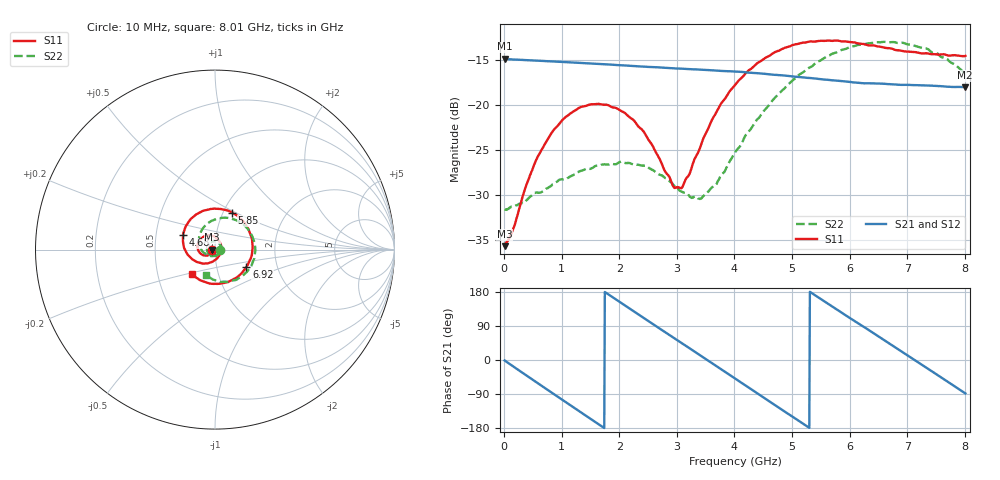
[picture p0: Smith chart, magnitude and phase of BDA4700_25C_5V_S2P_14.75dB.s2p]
!Agilent Technologies,E5071B,MY42404982,A.09.10
!Date: Mon Oct 20 13:33:35 2025
!Data & Calibration Information:
!Freq	S11:SOLT2(ON)	S21:SOLT2(ON)	S12:SOLT2(ON)	S22:SOLT2(ON)
# Hz S RI R 50
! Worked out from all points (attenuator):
!   801 points, 10 MHz to 8.01 GHz, reference 50 ohm
!   highest |S21| = -14.85 dB at 10 MHz (marker M1); lowest = -18.0 dB at 8 GHz (marker M2)
!   lowest |S11| = -35.7 dB at 10 MHz (marker M3), VSWR 1.03, Z = 48.4 - j0.117 ohm
!   |S11| at or under -10 dB: start of sweep to end of sweep
!   |S22| runs from -31.7 to -13.0 dB; largest |S21 - S12| = 0.0014
!   S11 on the Smith chart (normalised r, x): 10 MHz: 0.97, -0.00; 4.68 GHz: 0.69, +0.11; 5.85 GHz: 1.10, +0.48; 6.92 GHz: 1.39, -0.28; 8.01 GHz: 0.75, -0.21
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1e7  -0.0164 -0.00121  0.1809 -0.00401  0.1809 -0.00411  0.0263 -0.00101
1.5e8  -0.0176 -0.00972  0.1725 -0.0494  0.1725 -0.0495  0.0263 -0.00743
3.9e8  -0.0265 -0.0247  0.1344 -0.1166  0.1343 -0.1167  0.0207 -0.0211
6.3e8  -0.0434 -0.0333  0.0725 -0.1608  0.0724 -0.1609  0.00968 -0.0312
1.01e9  -0.079 -0.0235  -0.0446 -0.1681  -0.0446 -0.1681  -0.0188 -0.0339
1.35e9  -0.0976 0.00893  -0.1308 -0.1109  -0.1309 -0.111  -0.0406 -0.0146
1.72e9  -0.0855 0.0529  -0.1687 -0.00723  -0.1689 -0.00732  -0.0436 0.0168
2.08e9  -0.0468 0.0784  -0.1377 0.0933  -0.1377 0.0934  -0.0241 0.0413
2.68e9  0.0255 0.0448  0.0134 0.1616  0.0133 0.1616  0.0241 0.0335
2.94e9  0.0344 0.00725  0.0823 0.1375  0.0824 0.1374  0.033 0.0145
3.08e9  0.0313 -0.0145  0.113 0.1125  0.1124 0.1129  0.033 0.00166
3.43e9  -0.00419 -0.0614  0.1552 0.0267  0.1552 0.0266  0.0158 -0.0259
4.01e9  -0.1134 -0.0621  0.1013 -0.1156  0.1014 -0.1154  -0.0453 -0.0297
4.68e9  -0.1784 0.0797  -0.066 -0.132  -0.0658 -0.1323  -0.0898 0.0599
5.35e9  -0.0581 0.2183  -0.1407 0.00998  -0.1408 0.00962  -0.00632 0.1645
5.85e9  0.0957 0.2055  -0.0803 0.1099  -0.0801 0.11  0.1176 0.1644
6.25e9  0.1861 0.1146  0.0067 0.1321  0.00809 0.1321  0.1984 0.0912
6.68e9  0.2057 -0.025  0.0935 0.0915  0.0937 0.0914  0.222 -0.0251
6.92e9  0.1751 -0.0966  0.1212 0.0462  0.1211 0.0456  0.2032 -0.09
7.47e9  0.0268 -0.1901  0.1062 -0.0715  0.1061 -0.0718  0.0816 -0.1787
8e9  -0.1262 -0.1386  0.00638 -0.1257  0.0064 -0.126  -0.046 -0.1428
8.01e9  -0.1289 -0.137  0.00394 -0.1259  0.00423 -0.126  -0.0483 -0.1411
